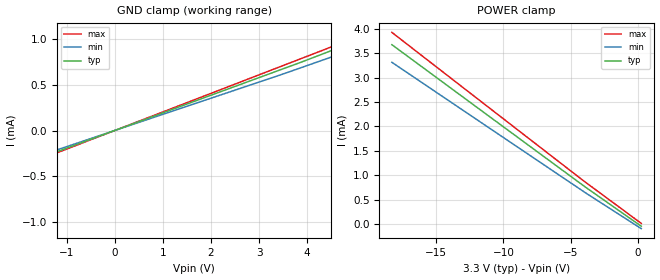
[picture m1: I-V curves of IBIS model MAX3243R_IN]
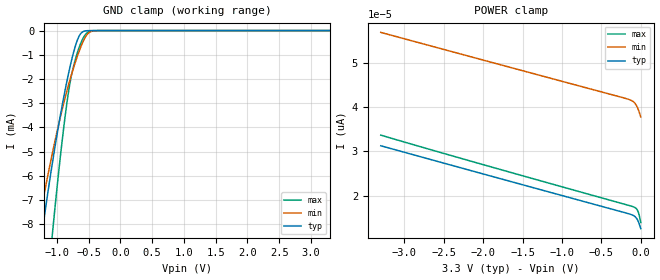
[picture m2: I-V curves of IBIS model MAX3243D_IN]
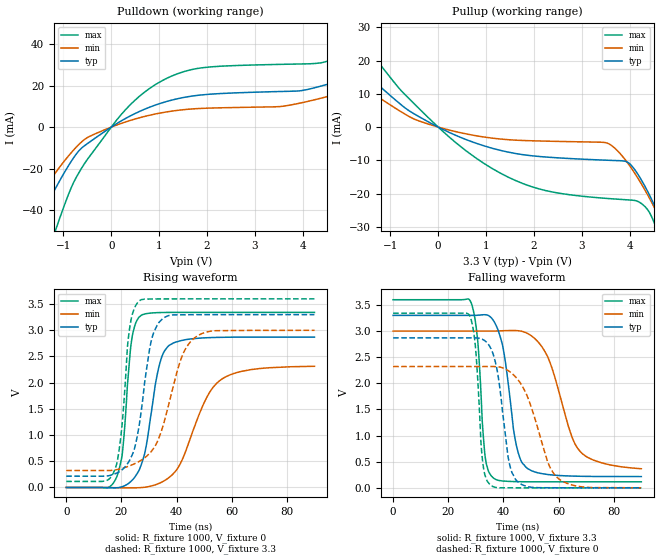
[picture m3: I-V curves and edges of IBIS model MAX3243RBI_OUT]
| TEXAS INSTRUMENTS INCORPORATED
| Standard Linear and Logic Group
| IBIS Model of MAX3243
| 3-V TO 5.5-V MULTICHANNEL RS-232 LINE DRIVER/RECEIVER WITH +-15 kV ESD
| (HBM) PROTECTION
| This file contains package information for the following:
|  SSOP 28-pin (DB) package as [Component] MAX3243C_DB
|  SOIC 28-pin (DW) package as [Component] MAX3243C_DW
|  TSSOP 28-pin (PW) package as [Component] MAX3243C_PW
| This device can be powered at the following Vccs:
|  3.3 volt Vcc
| This file provides unique models under the [Model Selector] for each Vcc.
| For operation at a specific Vcc, select the appropriate model after each
| [Model Selector] keyword.
[IBIS Ver]   3.2
[Comment char]  |_char
[File Name]   max3243.ibs
[File Rev]   1.1 | c_die
[Date]   June 18, 2001
[Source]   Data created from TI-SPICE simulations at TI-SLL.
[Notes]   The following is an IBIS list for the MAX3243C.
   Please contact sllibis@ti.com with questions and
   comments concerning SLL IBIS models.
   -We violated the sweep range for receiver input and
   driver output assuming that there will be no reflection
   issue in practice.
   - This model has data only for 3.3 V VCC
   - Since the receiver of RS-232 has no Vinl and Vinh, we
   omitted those parameters
   - FILE REV HISTORY
   - 1.0   RELEASE IBIS FILE ON 06/18/2001
   - 1.1   ADDED PW PACKAGE ON 01/19/2004
[Disclaimer] Property of Texas Instruments Incorporated.  Unauthorized
   reproduction and/or distribution is strictly prohibited.
   This product is protected under copyright law.
   Created  2001, (C) Copyright  2001, Texas Instruments
   Incorporated, All Rights Reserved
   UNLESS THERE IS A SIGNED, WRITTEN AGREEMENT TO THE
   CONTRARY, TEXAS INSTRUMENTS (TI) IS PROVIDING THE IBIS
   MODELS  AND WITHOUT ANY WARRANTY, EXPRESSED OR
   IMPLIED.  TI assumes no liability for:
   1) the accuracy of the IBIS models provided to your
   company;
   2) the proper functioning of these IBIS Models in your
   design or for any resulting applications; or
   3) infringement of patents, copyrights or intellectual
   property rights resulting from your use of these IBIS
   models.
   TI provides IBIS Models as a service to our customers.
   You and your company shall not distribute, sell or give
   these models to anyone else without prior written
   permission from TI.
   TI reserves the right to make changes to our products or
   to discontinue any semiconductor product or service
   without notice, and advises our customers to obtain the
   latest version of relevant information to verify, before
   placing orders, that the information being relied on is
   current.
   Please be aware that your receipt and use of the IBIS
   information provided shall serve as acceptance of these
   terms and conditions.  If you do not accept these terms,
   you should return or destroy the IBIS models and any
   other accompanying information immediately.
| Component MAX3243C_DB 28-pin SSOP
[Component]   MAX3243C_DB
[Manufacturer]   Texas Instruments, Inc.
[Package]
|   typ   min   max
R_pkg   3.400e-02   2.800e-02   3.900e-02
L_pkg   3.404e-09   2.704e-09   4.545e-09
C_pkg   4.280e-13   2.990e-13   5.710e-13
[Pin]   signal_name   model_name   R_pin   L_pin   C_pin
1   C2+   NC   3.800e-02   4.545e-09   5.640e-13
2   C2-   NC   3.900e-02   4.133e-09   5.710e-13
3   VMINUS   NC   3.500e-02   3.598e-09   4.890e-13
4   RIN1   MAX3243R_IN   2.800e-02   3.087e-09   4.080e-13
5   RIN2   MAX3243R_IN   3.200e-02   2.990e-09   3.490e-13
6   RIN3   MAX3243R_IN   3.200e-02   2.774e-09   3.180e-13
7   RIN4   MAX3243R_IN   3.100e-02   2.704e-09   2.990e-13
8   RIN5   MAX3243R_IN   3.100e-02   2.704e-09   2.990e-13
9   DOUT1   MAX3243D_OUT   3.200e-02   2.774e-09   3.180e-13
10   DOUT2   MAX3243D_OUT   3.200e-02   2.990e-09   3.490e-13
11   DOUT3   MAX3243D_OUT   2.800e-02   3.087e-09   4.080e-13
12   DIN3   MAX3243D_IN   3.500e-02   3.598e-09   4.890e-13
13   DIN2   MAX3243D_IN   3.900e-02   4.133e-09   5.710e-13
14   DIN1   MAX3243D_IN   3.800e-02   4.545e-09   5.640e-13
15   ROUT5   MAX3243R_OUT   3.800e-02   4.545e-09   5.640e-13
16   ROUT4   MAX3243R_OUT   3.900e-02   4.133e-09   5.710e-13
17   ROUT3   MAX3243R_OUT   3.500e-02   3.597e-09   4.890e-13
18   ROUT2   MAX3243R_OUT   2.800e-02   3.087e-09   4.080e-13
19   ROUT1   MAX3243R_OUT   3.200e-02   2.990e-09   3.490e-13
20   ROUT2B   MAX3243RBI_OUT   3.100e-02   2.774e-09   3.180e-13
21   INVALID   MAX3243RBI_OUT   3.100e-02   2.704e-09   2.990e-13
22   FORCEOFFB  MAX3243F_IN   3.100e-02   2.704e-09   2.990e-13
23   FORCEON   MAX3243F_IN   3.200e-02   2.774e-09   3.180e-13
24   C1-   NC   3.200e-02   2.990e-09   3.490e-13
25   GND   GND   2.800e-02   3.087e-09   4.080e-13
26   VCC   POWER   3.500e-02   3.598e-09   4.890e-13
27   VPLUS   NC   3.900e-02   4.133e-09   5.710e-13
28   C1+   NC   3.800e-02   4.545e-09   5.640e-13
| Component MAX3243C_DW 28-pin SOIC
[Component]   MAX3243C_DW
[Manufacturer]   Texas Instruments, Inc.
[Package]
|   typ   min   max
R_pkg   3.700e-02   3.100e-02   4.600e-02
L_pkg   5.147e-09   3.554e-09   7.390e-09
C_pkg   8.040e-13   3.820e-13   1.314e-12
[Pin]   signal_name   model_name   R_pin   L_pin   C_pin
1   C2+   NC   4.500e-02   7.390e-09   1.122e-12
2   C2-   NC   4.300e-02   6.387e-09   1.048e-12
3   VMINUS   NC   3.800e-02   5.461e-09   8.240e-13
4   RIN1   MAX3243R_IN   3.700e-02   4.759e-09   5.730e-13
5   RIN2   MAX3243R_IN   3.100e-02   4.604e-09   5.090e-13
6   RIN3   MAX3243R_IN   3.200e-02   3.891e-09   4.580e-13
7   RIN4   MAX3243R_IN   3.400e-02   3.554e-09   3.820e-13
8   RIN5   MAX3243R_IN   3.400e-02   3.555e-09   3.820e-13
9   DOUT1   MAX3243D_OUT   3.200e-02   3.891e-09   4.580e-13
10   DOUT2   MAX3243D_OUT   3.100e-02   4.604e-09   5.090e-13
11   DOUT3   MAX3243D_OUT   3.300e-02   4.744e-09   5.730e-13
12   DIN3   MAX3243D_IN   3.600e-02   5.454e-09   8.240e-13
13   DIN2   MAX3243D_IN   4.200e-02   6.382e-09   1.049e-12
14   DIN1   MAX3243D_IN   4.600e-02   7.383e-09   1.074e-12
15   ROUT5   MAX3243R_OUT   4.600e-02   7.383e-09   1.266e-12
16   ROUT4   MAX3243R_OUT   4.200e-02   6.382e-09   1.262e-12
17   ROUT3   MAX3243R_OUT   3.600e-02   5.454e-09   1.037e-12
18   ROUT2   MAX3243R_OUT   3.300e-02   4.744e-09   7.870e-13
19   ROUT1   MAX3243R_OUT   3.100e-02   4.604e-09   7.230e-13
20   ROUT2B   MAX3243RBI_OUT   3.200e-02   3.891e-09   6.710e-13
21   INVALID   MAX3243RBI_OUT   3.400e-02   3.554e-09   5.960e-13
22   FORCEOFFB  MAX3243F_IN   3.400e-02   3.554e-09   5.960e-13
23   FORCEON   MAX3243F_IN   3.200e-02   3.891e-09   6.710e-13
24   C1-   NC   3.100e-02   4.604e-09   7.230e-13
25   GND   GND   3.700e-02   4.759e-09   7.870e-13
26   VCC   POWER   3.800e-02   5.461e-09   1.037e-12
27   VPLUS   NC   4.300e-02   6.387e-09   1.261e-12
28   C1+   NC   4.500e-02   7.390e-09   1.314e-12
| Component MAX3243C_PW 28-pin TSSOP
[Component]   MAX3243C_PW
[Manufacturer]   Texas Instruments, Inc.
[Package]
|   typ   min   max
R_pkg   2.300e-02   1.900e-02   3.000e-02
L_pkg   1.781e-09   1.295e-09   2.916e-09
C_pkg   1.390e-13   7.700e-14   3.160e-13
[Pin]   signal_name   model_name   R_pin   L_pin   C_pin
1   C2+   NC   3.000e-02   2.916e-09   3.160e-13
2   C2-   NC   2.900e-02   2.409e-09   1.910e-13
3   VMINUS   NC   2.500e-02   1.805e-09   1.400e-13
4   RIN1   MAX3243R_IN   2.000e-02   1.336e-09   9.200e-14
5   RIN2   MAX3243R_IN   2.000e-02   1.329e-09   8.000e-14
6   RIN3   MAX3243R_IN   2.100e-02   1.360e-09   7.900e-14
7   RIN4   MAX3243R_IN   2.100e-02   1.359e-09   7.900e-14
8   RIN5   MAX3243R_IN   2.100e-02   1.343e-09   7.800e-14
9   DOUT1   MAX3243D_OUT   2.000e-02   1.327e-09   7.800e-14
10   DOUT2   MAX3243D_OUT   2.100e-02   1.345e-09   8.000e-14
11   DOUT3   MAX3243D_OUT   2.000e-02   1.335e-09   9.200e-14
12   DIN3   MAX3243D_IN   2.500e-02   1.799e-09   1.420e-13
13   DIN2   MAX3243D_IN   2.600e-02   2.338e-09   1.890e-13
14   DIN1   MAX3243D_IN   2.800e-02   2.878e-09   3.140e-13
15   ROUT5   MAX3243R_OUT   3.000e-02   2.910e-09   3.140e-13
16   ROUT4   MAX3243R_OUT   2.900e-02   2.431e-09   1.910e-13
17   ROUT3   MAX3243R_OUT   2.700e-02   1.903e-09   1.450e-13
18   ROUT2   MAX3243R_OUT   1.900e-02   1.319e-09   9.100e-14
19   ROUT1   MAX3243R_OUT   1.900e-02   1.313e-09   7.900e-14
20   ROUT2B   MAX3243RBI_OUT   2.000e-02   1.327e-09   7.800e-14
21   INVALID   MAX3243RBI_OUT   2.000e-02   1.327e-09   7.800e-14
22   FORCEOFFB  MAX3243F_IN   1.900e-02   1.295e-09   7.700e-14
23   FORCEON   MAX3243F_IN   2.000e-02   1.327e-09   7.800e-14
24   C1-   NC   2.000e-02   1.328e-09   8.000e-14
25   GND   GND   2.000e-02   1.335e-09   9.200e-14
26   VCC   POWER   2.700e-02   1.894e-09   1.450e-13
27   VPLUS   NC   2.700e-02   2.397e-09   1.900e-13
28   C1+   NC   2.900e-02   2.892e-09   3.140e-13
| Models and submodels in the file (6): MAX3243R_IN (Input), MAX3243D_IN (Input), MAX3243F_IN (Input), MAX3243RBI_OUT (Output), MAX3243R_OUT (3-state), MAX3243D_OUT (3-state)
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| Model MAX3243R_IN
[Model]   MAX3243R_IN
Model_type  Input
Vinl = 0.8
Vinh = 2.0
| variable   typ   min   max
C_comp   0.00pF   0.00pF   0.00pF
[Model Spec]
| variable   typ   min   max
Vinl+   1.1   NA   NA
Vinl-   0.6   NA   NA
Vinh+   2.4   NA   NA
Vinh-   1.6   NA   NA
[Temperature Range]   40   100   -40
| Ambient temperature   25   85   -40
[Voltage range]   3.3   3   3.6
[GND Clamp]
| MAX3243R_IN_33
|   Voltage   I(typ)   I(min)   I(max)
-15V      -3.025mA   -2.768mA   -3.187mA
-6.4V     -1.281mA   -1.172mA   -1.35mA
-6V       -1.2mA     -1.098mA   -1.264mA
-5.6V     -1.119mA   -1.024mA   -1.179mA
-5.2V     -1.038mA   -949.4uA   -1.093mA
-1.4V     -271.4uA   -248.5uA   -285.7uA
3.4V      657.7uA    602.3uA    692.3uA
5.25V     1.028mA    944.6uA    1.077mA
5.65V     1.109mA    1.019mA    1.163mA
6.45V     1.271mA    1.167mA    1.333mA
25V       5.038mA    4.617mA    5.297mA
[POWER Clamp]
| MAX3243R_IN_33
|   Voltage   I(typ)   I(min)   I(max)
-18.3V    3.676mA    3.315mA    3.929mA
-4.15V    804.9uA    684.9uA    906.9uA
-3.65V    706uA      593.3uA    804.3uA
250mV     -48.36uA   -97.41uA   10.18uA
[Model]   MAX3243D_IN
Model_type  Input
Vinl = 0.8
Vinh = 2.0
| variable   typ   min   max
C_comp   1.19pF   0.88pF   1.37pF
[Temperature Range]   40   100   -40
| Ambient temperature   25   85   -40
[Voltage range]   3.3   3   3.6
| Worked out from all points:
|   GND clamp passes 1 mA (typ) near -0.75 V on its own axis
[GND Clamp]
| MAX3243D_IN_33
|   Voltage   I(typ)   I(min)   I(max)
-3.3V     -67.98mA   -51.63mA   -103.5mA
-1.325V   -10.18mA   -8.567mA   -16.11mA
-1.29V    -9.491mA   -8.054mA   -14.98mA
-1.225V   -8.243mA   -7.13mA    -12.94mA
-1.065V   -5.412mA   -5.018mA   -8.304mA
-915mV    -3.102mA   -3.267mA   -4.558mA
-810mV    -1.722mA   -2.201mA   -2.458mA
-685mV    -463.1uA   -1.135mA   -993.7uA
-580mV    -36.07uA   -422.8uA   -290uA
-510mV    -3.311uA   -125.7uA   -63.81uA
-410mV    -77.71nA   -8.443uA   -1.584uA
3.3V      12.57pA    42.44pA    9.911pA
[POWER Clamp]
| MAX3243D_IN_33
|   Voltage   I(typ)   I(min)   I(max)
-3.3V     31.25pA    56.79pA    33.65pA
-2.045V   25.12pA    50.77pA    27.22pA
-170mV    16.02pA    41.8pA     17.9pA
-125mV    15.77pA    41.5pA     17.67pA
-95mV     15.55pA    41.18pA    17.5pA
-70mV     15.24pA    40.74pA    17.29pA
-50mV     14.82pA    40.17pA    16.96pA
-35mV     14.33pA    39.59pA    16.47pA
-25mV     13.91pA    39.11pA    15.96pA
-15mV     13.41pA    38.58pA    15.26pA
-48.03fV  12.57pA    37.72pA    13.95pA
[Model]   MAX3243RBI_OUT
Model_type  Output
Vref =   0.0
Rref =   3000
Cref =   150p
Vmeas =   1.5
| variable   typ   min   max
C_comp   3.21pF   2.18pF   5.20pF
| C_pullup   2.98pF   2.18pF   4.20pF
| C_pulldown   3.45pF   2.30pF   5.20pF
[Temperature Range]   40   100   -40
| Ambient temperature   25   85   -40
[Voltage range]   3.3   3   3.6
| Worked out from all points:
|   slope of the pulldown table from 0 to 0.495 V, typ, clamps not added: 75.8 ohm
|   slope of the pullup table from 0 to 0.495 V, typ, clamps not added: 152 ohm
|   rising waveform, R_fixture 1000, V_fixture 0: 20-80 % time 5.53ns typ, 11ns min, 3ns max; typ from 0 V to 2.87 V
|   falling waveform, R_fixture 1000, V_fixture 3.3: 20-80 % time 4.77ns typ, 9.17ns min, 2.49ns max; typ from 3.3 V to 0.216 V
|   rising waveform, R_fixture 1000, V_fixture 3.3: 20-80 % time 5.2ns typ, 8.83ns min, 3.22ns max; typ from 0.215 V to 3.3 V
|   falling waveform, R_fixture 1000, V_fixture 0: 20-80 % time 4.22ns typ, 8.55ns min, 2.26ns max; typ from 2.87 V to 0 V
[Pulldown]
| MAX3243RBI_OUT_33
|   Voltage   I(typ)   I(min)   I(max)
-3.3V     -150.1mA   -112.3mA   -224.8mA
-1.89V    -64.84mA   -48.09mA   -104.5mA
-1.565V   -48.09mA   -35.69mA   -78.88mA
-1.155V   -29.14mA   -21.7mA    -49.16mA
-725mV    -12.82mA   -9.525mA   -23.99mA
35mV      528.2uA    314.1uA    1.092mA
590mV     7.551mA    4.499mA    14.9mA
1.245V    12.9mA     7.634mA    24.44mA
2.06V     15.86mA    9.158mA    29mA
4.08V     18.06mA    12.27mA    30.48mA
6.095V    34.37mA    26.26mA    49.15mA
6.6V      39.72mA    30.61mA    56.18mA
[Pullup]
| MAX3243RBI_OUT_33
|   Voltage   I(typ)   I(min)   I(max)
-3.3V     39.89mA    30.01mA    57.27mA
-2.555V   29.8mA     22.1mA     43.59mA
-1.855V   20.49mA    14.94mA    30.66mA
-380mV    2.962mA    1.738mA    5.288mA
640mV     -4.077mA   -2.214mA   -7.763mA
1.62V     -7.962mA   -3.941mA   -16.11mA
3.57V     -9.996mA   -5.086mA   -21.51mA
4.055V    -11.9mA    -12.83mA   -21.99mA
4.31V     -17.65mA   -18.78mA   -23.82mA
4.575V    -25.5mA    -25.96mA   -31.23mA
4.75V     -31.52mA   -31.22mA   -38.81mA
6.6V      -123.9mA   -107mA     -164.6mA
[Ramp]
| MAX3243RBI_OUT_33
| variable   typ   min   max
dV/dt_r   1.73/5.71E-09   1.39/1.12E-08   2.01/3.08E-09
dV/dt_f   1.86/4.99E-09   1.59/9.25E-09   2.10/2.58E-09
R_load = 1000
[Rising Waveform]
| MAX3243RBI_OUT_33
R_fixture =   1000
C_fixture =   0
L_fixture =   0
V_fixture =   0
V_fixture_min = 0
V_fixture_max = 0
|   Time   V(typ)   V(min)   V(max)
0s        34.86nV    129.6nV    -2.176nV
18.31ns   -5.763mV   -5.048mV   201.1mV
20.35ns   15.41mV    -5.94mV    659.6mV
23.75ns   131.3mV    -6.584mV   2.826V
27.18ns   429.6mV    -2.175mV   3.286V
29.04ns   807.3mV    8.856mV    3.318V
33.51ns   2.28V      75.19mV    3.338V
37.36ns   2.714V     194.3mV    3.341V
55.82ns   2.866V     2.046V     3.342V
90ns      2.87V      2.313V     3.342V
[Falling Waveform]
| MAX3243RBI_OUT_33
R_fixture =   1000
C_fixture =   0
L_fixture =   0
V_fixture =   3.3
V_fixture_min = 3
V_fixture_max = 3.6
|   Time   V(typ)   V(min)   V(max)
0s        3.3V       3V         3.6V
27.96ns   3.3V       3V         3.579V
30.71ns   3.303V     3V         2.797V
33.43ns   3.313V     3V         578.1mV
36.5ns    3.191V     3V         182.2mV
44.72ns   803.7mV    3.009V     118.7mV
48.1ns    398.3mV    2.971V     116.4mV
55.95ns   256.2mV    2.519V     115.3mV
67.75ns   221.5mV    699.8mV    115.2mV
90ns      215.6mV    365.4mV    115.2mV
[Rising Waveform]
| MAX3243RBI_OUT_33
R_fixture =   1000
C_fixture =   0
L_fixture =   0
V_fixture =   3.3
V_fixture_min = 3
V_fixture_max = 3.6
|   Time   V(typ)   V(min)   V(max)
0s        215.4mV    323.9mV    115.2mV
17.47ns   257mV      331.8mV    322.6mV
20ns      328.4mV    361.8mV    1.074V
22.99ns   520.4mV    413.5mV    3.043V
26.65ns   1.258V     503.9mV    3.568V
30.78ns   2.787V     684.2mV    3.597V
35.51ns   3.243V     1.253V     3.599V
42.01ns   3.296V     2.507V     3.6V
47.45ns   3.298V     2.89V      3.6V
90ns      3.3V       3V         3.6V
[Falling Waveform]
| MAX3243RBI_OUT_33
R_fixture =   1000
C_fixture =   0
L_fixture =   0
V_fixture =   0
V_fixture_min = 0
V_fixture_max = 0
|   Time   V(typ)   V(min)   V(max)
0s        2.87V      2.321V     3.342V
27.7ns    2.87V      2.321V     3.297V
29.84ns   2.869V     2.321V     2.703V
32.5ns    2.839V     2.321V     482.5mV
35.39ns   2.671V     2.322V     50.07mV
38ns      2.165V     2.316V     675.1uV
41.96ns   513.3mV    2.234V     1.094mV
44.93ns   127mV      2.09V      515.4uV
59.39ns   1.43mV     202.5mV    59.37uV
90ns      24.56uV    1.237mV    3.863uV
